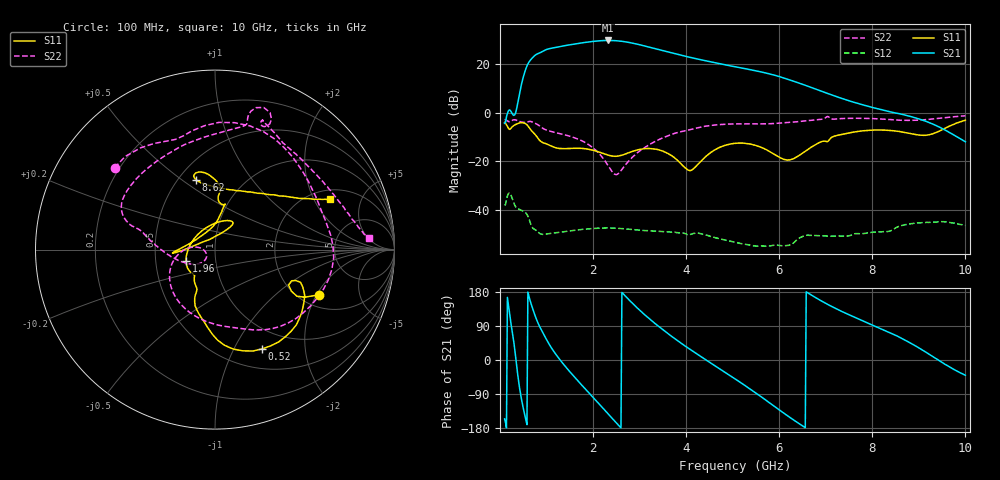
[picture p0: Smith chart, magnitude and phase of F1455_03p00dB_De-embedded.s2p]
! Integrated Device Technology
! Corporate Headquarters
! 6024 Silver Creek Valley Road
! San Jose, CA 95138  USA
! Phone:  1-408-284-8200
! Toll Free:  1-800-223-1366
! Webpage:  http://www.idt.com/
! Timing and RF Division
! 515 Groton Road, Suite 102
! Westford, MA 01886-6024
! Device:  F1455
! Description: 6-bit 0.5 dB Transmit Variable Gain Amplifier
! Frequency:  1400.0 -  2300.00 MHz
! Package:  6x6 mm Thin QFN Plastic Package: 28 pin
! State:  6
! Atten State:  3.0 dB
! Voltage:  +5.00 Volts
! Current:  215.388 mA
! Data:  The device was measured on a the F1455 evaluation board which has
!  individual transmission lines to the RF pins.  Data was collected
!  using a calibrated network analyzer.  The evaluation board was
!  de-embedded using a TRL calibration technique.
!  The reference plane is the edge of the package pin.
!  Pin  1 = CSb
!  Pin  2 = DATA
!  Pin  3 = CLK
!  Pin  4 = RSET
!  Pin  5 = GND
!  Pin  6 = RFIN  = Port 1
!  Pin  7 = GND
!  Pin  8 = NC
!  Pin  9 = NC
!  Pin 10 = NC
!  Pin 11 = NC
!  Pin 12 = NC
!  Pin 13 = NC
!  Pin 14 = /STBY
!  Pin 15 = GND
!  Pin 16 = RFOUT  = Port 2
!  Pin 17 = GND
!  Pin 18 = NC
!  Pin 19 = NC
!  Pin 20 = NC
!  Pin 21 = GND
!  Pin 22 = NC
!  Pin 23 = GND
!  Pin 24 = NC
!  Pin 25 = NC
!  Pin 26 = NC
!  Pin 27 = GND
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# GHz S dB R 50
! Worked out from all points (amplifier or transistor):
!   496 points, 100 MHz to 10 GHz, reference 50 ohm
!   highest |S21| = 29.8 dB at 2.32 GHz (marker M1)
!   |S21| within 3 dB of that: 1.159 GHz to 3.257 GHz (2.098 GHz wide, 95 % of centre)
!   unconditionally stable (mu >= 1): start of sweep to end of sweep
!   at 1.74 GHz: K = 4.22, MAG = 29.2 dB, |S12| = -48.1 dB
!   at 5.06 GHz: K = 16.39, MAG = 21.0 dB, |S12| = -53.4 dB
!   at 10 GHz: K = 53.67, MAG = -3.1 dB, |S12| = -46.4 dB
!   S11 on the Smith chart (normalised r, x): 100 MHz: 2.50, -2.10; 520 MHz: 0.73, -1.30; 1.96 GHz: 0.72, -0.09; 8.62 GHz: 0.61, +0.57; 10 GHz: 2.44, +2.71
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0.1  -3.98 -23.5  -4.34 -155.5  -38.18 40.6  -2.83 140.8
0.4  -4.34 -39.3  5.82 -55.8  -39.66 -112.5  -3.43 50.4
0.52  -4.26 -64.6  15.94 -138.0  -40.76 -151.2  -3.99 23.7
0.7  -7.88 -98.9  22.67 136.4  -47.36 154.1  -3.84 -20.7
0.82  -10.62 -112.6  24.37 96.7  -49.20 137.6  -5.01 -49.6
0.96  -12.60 -116.1  25.72 63.3  -50.06 124.2  -6.83 -73.8
1.14  -14.04 -125.6  26.70 25.7  -49.58 101.6  -7.92 -97.7
1.34  -14.76 -129.9  27.44 -7.3  -49.09 79.8  -8.85 -120.8
1.54  -14.67 -136.1  28.11 -36.5  -48.60 61.7  -9.91 -140.2
1.76  -14.68 -146.1  28.77 -66.6  -48.05 44.6  -11.56 -158.6
1.96  -15.23 -159.0  29.29 -93.2  -47.73 30.9  -13.87 -173.5
2.32  -17.44 159.3  29.77 -141.6  -47.46 7.4  -21.72 173.6
2.6  -17.59 110.2  29.46 -179.1  -47.71 -8.8  -23.88 -138.2
2.9  -15.60 74.1  28.45 143.2  -48.21 -23.3  -17.34 -143.2
3.4  -15.22 55.3  26.07 89.6  -48.83 -42.7  -11.21 -176.1
4.08  -23.88 114.8  22.81 28.4  -50.24 -65.9  -7.00 164.8
5.06  -12.57 -175.3  18.91 -50.6  -53.36 -102.1  -4.60 148.5
5.94  -17.64 160.3  15.24 -126.2  -54.56 -109.4  -4.37 108.9
6.7  -14.06 81.3  10.33 170.7  -50.46 -136.4  -3.13 78.2
8.36  -7.27 105.6  0.46 72.8  -48.87 170.8  -2.78 62.1
8.62  -7.86 105.3  -0.56 57.9  -46.51 164.3  -3.10 54.0
10  -3.08 23.8  -11.98 -40.3  -46.43 84.6  -1.29 4.5
